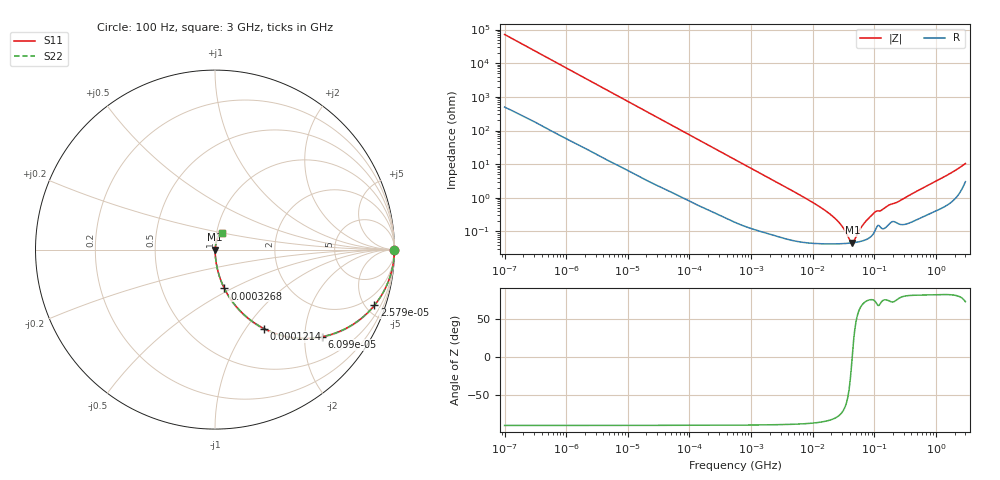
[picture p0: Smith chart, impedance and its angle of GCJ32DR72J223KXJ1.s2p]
!Murata Part Number: GCJ32DR72J223KXJ1
!These Parameters are Measured in Series Mode Connection
!Data Generated on Mar 13, 2026
!  o--ll--o
!Port1  Port2
!  o------o
!Operation Temp=25[degC], DC Bias Voltage=0[V]
!Freq. Start=100[Hz] Stop=3[GHz] 401[Steps]
# Hz S RI R 50
!Freq.(Hz) S11(Real) S11(Imag) S21(Real) S21(Imag) S12(Real) S12(Imag) S22(Real) S22(Imag)
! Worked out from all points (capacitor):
!   401 points, 100 Hz to 3 GHz, reference 50 ohm
!   read as one part in series: C = 22.2 nF near 109 Hz
!   lowest |Z| = 46.1 mohm at 44.18 MHz (marker M1)
!   series resonance near 43.66 MHz, so ESL is about 600 pH
!   S11 on the Smith chart (normalised r, x): 100 Hz: open; 25.79 kHz: 1.05, -5.71; 60.99 kHz: 1.02, -2.43; 121.4 kHz: 1.01, -1.22; 326.8 kHz: 1.01, -0.46; 3 GHz: 1.06, +0.20
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100  1 -0.0014  1.17e-05 0.0014  1.17e-05 0.0014  1 -0.0014
1788  0.9992 -0.0246  0.00081 0.0246  0.00081 0.0246  0.9992 -0.0246
8066  0.9871 -0.1088  0.0129 0.1088  0.0129 0.1088  0.9871 -0.1088
25785  0.8884 -0.3103  0.1116 0.3103  0.1116 0.3103  0.8884 -0.3103
31977  0.8392 -0.3627  0.1608 0.3627  0.1608 0.3627  0.8392 -0.3627
60986  0.5945 -0.4859  0.4055 0.4859  0.4055 0.4859  0.5945 -0.4859
121426  0.2747 -0.441  0.7253 0.441  0.7253 0.441  0.2747 -0.441
194955  0.1304 -0.331  0.8696 0.331  0.8696 0.331  0.1304 -0.331
326774  0.0523 -0.2164  0.9477 0.2164  0.9477 0.2164  0.0523 -0.2164
547723  0.0202 -0.1341  0.9798 0.1341  0.9798 0.1341  0.0202 -0.1341
1677156  0.00293 -0.0449  0.9971 0.0449  0.9971 0.0449  0.00293 -0.0449
9794414  0.000499 -0.00742  0.9995 0.00742  0.9995 0.00742  0.000499 -0.00742
2.418395e7  0.000432 -0.0022  0.9996 0.0022  0.9996 0.0022  0.000432 -0.0022
3.131008e7  0.000436 -0.00119  0.9996 0.00119  0.9996 0.00119  0.000436 -0.00119
4.0536e7  0.000451 -0.000261  0.9995 0.000261  0.9995 0.000261  0.000451 -0.000261
4.418008e7  0.000458 4.29e-05  0.9995 -4.29e-05  0.9995 -4.29e-05  0.000458 4.29e-05
6.508213e7  0.000529 0.00147  0.9995 -0.00147  0.9995 -0.00147  0.000529 0.00147
8.79653e7  0.000709 0.0028  0.9993 -0.0028  0.9993 -0.0028  0.000709 0.0028
1.044919e8  0.00114 0.00369  0.9989 -0.00369  0.9989 -0.00369  0.00114 0.00369
1.751444e8  0.00171 0.00591  0.9983 -0.00591  0.9983 -0.00591  0.00171 0.00591
2.471375e8  0.00174 0.00756  0.9983 -0.00756  0.9983 -0.00756  0.00174 0.00756
3e9  0.0383 0.0934  0.9617 -0.0934  0.9617 -0.0934  0.0383 0.0934
